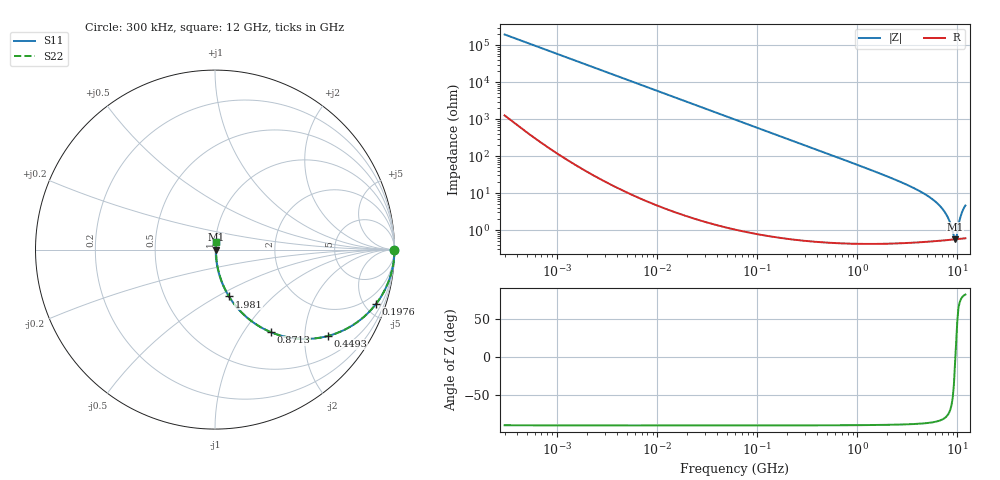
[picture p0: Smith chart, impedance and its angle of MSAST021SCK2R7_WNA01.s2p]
! MSAST021SCK2R7_WNA01  S-PARAMETER MODEL  ( General Type )
! Model Generated by TAIYO YUDEN Corporation (http://www.ty-top.com)
! Version 2.0
! TAIYO YUDEN Control No. 181101
! Copyright(c) 2015 TAIYO YUDEN CO.,LTD. All Rights Reserved.
! Product Description (link to TY-COMPAS)
! https://ds.yuden.co.jp/TYCOMPAS/or/detail?pn=MSAST021SCK2R7BWNA01&u=M
! Products Name : Multilayer Ceramic Capacitors
! Characteristics :
!  Capacitance : 2.7 pF , Rated Voltage : 25V , TCC : CK / C0K
!  Case Size : 0.25 x 0.125 / 0.0098 x 0.0049 [mm/inch] , Thickness : 0.125 / 0.0049 [mm/inch]
!  (Conditions: Temperature = 25 degC , DC Bias Current/Voltage = 0A / 0V)
! External Node Assignments :
!  1  o---| |---o  2
! GND o---------o GND
! Frequency Range : 0.3MHz  -  12000MHz  [ 401 STEP ]
# MHz S RI R 50
! Freq[MHz].  S11 Real  S11 Imag  S21 Real  S21 Imag  S12 Real  S12 Imag  S22 Real  S22 Imag
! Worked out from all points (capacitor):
!   401 points, 300 kHz to 12 GHz, reference 50 ohm
!   read as one part in series: C = 2.7 pF near 316.3 kHz
!   lowest |Z| = 568 mohm at 9.454 GHz (marker M1)
!   series resonance near 9.533 GHz, so ESL is about 100 pH
!   S11 on the Smith chart (normalised r, x): 300 kHz: open; 197.6 MHz: 1.01, -5.96; 449.3 MHz: 1.01, -2.62; 871.3 MHz: 1.01, -1.34; 1.981 GHz: 1.01, -0.57; 12 GHz: 1.01, +0.09
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0.3  1 -0.000509  3.53e-06 0.000509  3.53e-06 0.000509  1 -0.000509
1.769972  1 -0.003  1.31e-05 0.003  1.31e-05 0.003  1 -0.003
10.44266  0.9997 -0.0177  0.000328 0.0177  0.000328 0.0177  0.9997 -0.0177
60  0.9896 -0.1007  0.0104 0.1007  0.0104 0.1007  0.9896 -0.1007
197.6437  0.8984 -0.3012  0.1016 0.3012  0.1016 0.3012  0.8984 -0.3012
353.9943  0.7338 -0.4405  0.2662 0.4405  0.2662 0.4405  0.7338 -0.4405
449.3064  0.631 -0.4808  0.369 0.4808  0.369 0.4808  0.631 -0.4808
617.4538  0.4748 -0.497  0.5252 0.497  0.5252 0.497  0.4748 -0.497
871.3074  0.3115 -0.4599  0.6885 0.4599  0.6885 0.4599  0.3115 -0.4599
1296.429  0.1684 -0.3695  0.8316 0.3695  0.8316 0.3695  0.1684 -0.3695
1980.756  0.0783 -0.2613  0.9217 0.2613  0.9217 0.2613  0.0783 -0.2613
2088.533  0.0708 -0.2486  0.9292 0.2486  0.9292 0.2486  0.0708 -0.2486
3944.255  0.0195 -0.1208  0.9805 0.1208  0.9805 0.1208  0.0195 -0.1208
6026.253  0.00837 -0.0578  0.9916 0.0578  0.9916 0.0578  0.00837 -0.0578
6879.757  0.00679 -0.0404  0.9932 0.0404  0.9932 0.0404  0.00679 -0.0404
7648.807  0.00601 -0.027  0.994 0.027  0.994 0.027  0.00601 -0.027
8281.503  0.00568 -0.0171  0.9943 0.0171  0.9943 0.0171  0.00568 -0.0171
9207.246  0.00556 -0.00409  0.9944 0.00409  0.9944 0.00409  0.00556 -0.00409
9454.42  0.00558 -0.000887  0.9944 0.000887  0.9944 0.000887  0.00558 -0.000887
9968.853  0.0057 0.00625  0.9943 -0.00625  0.9943 -0.00625  0.0057 0.00625
11083.22  0.00669 0.0291  0.9933 -0.0291  0.9933 -0.0291  0.00669 0.0291
12000  0.00802 0.0451  0.992 -0.0451  0.992 -0.0451  0.00802 0.0451
